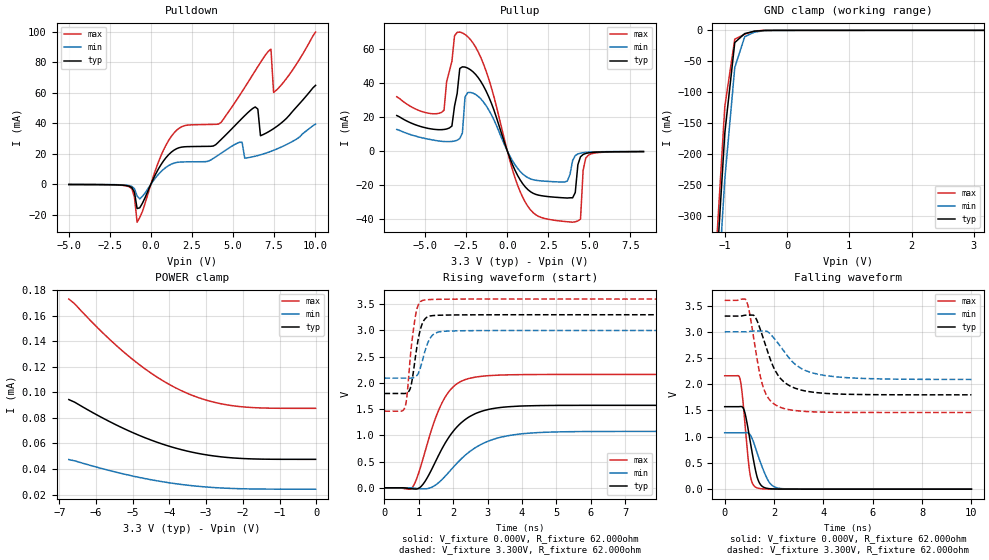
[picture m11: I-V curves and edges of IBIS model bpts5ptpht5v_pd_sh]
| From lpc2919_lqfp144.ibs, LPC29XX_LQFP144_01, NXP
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| |   Rev 0.20 IBIS Model Design Automation Generation   |
| |   N O N - S I L I C O N   C O R R E L A T E D   |
| |   This IBIS [Model] is pre-Beta tactical support   |
| |  Note: this IBIS [Model] contains clamp curves generated   |
| |   through simulation which should not be relied upon   |
| Pccmos14 hliolib_nlm 4.0.1
|   0.18 um 3.3V pad library
|   six level metal
|   dual oxide
|   single threshold voltage
|   nominal line mixed supply
|   parasitic extracted netlists
| Process block c14
| bpts5ptpht5v
|   Bidirectional Pad 3v3
|   3state Output
|   Plain Input
|   1ns Slew Rate control
|   CMOS
|   Programmable between
|   - (p1=0, p2=1) plain input
|   - (p1=0, p2=0) with Pull Up
|   - (p1=1, p2=1) with Pull Down
|   - (p1=1, p2=0) with Repeater
|   Characterized at Core 1.8V and I/O 3.3V
| Pull Down Mode (p1=1, p2=1)
[Model]   bpts5ptpht5v_pd_sh | of bpts5ptpht5v
Model_type   I/O
Polarity   Non-Inverting
Enable   Active-Low
|  Reciever Thresholds
Vinl   = 0.99V
Vinh   = 2.31V
| AC Test Load Conditions
Vref   = 0
Cref   = 1.2e-11
Rref   = 1000000000
Vmeas   = 1.65
| [Process Range]   typical   min   max
| C_comp edge width   400.000ps   400.000ps   400.000ps
| C_comp Tstrobe   40.000fs   40.000fs   40.000fs
C_comp   2.521pF   2.386pF   2.657pF
[Temperature Range]   25   125   -40
[Voltage Range]   3.30V   3.00V   3.60V
[GND Clamp Reference]   0.00V   0.00V   0.00V
[Pulldown Reference]   0.00V   0.00V   0.00V
[POWER Clamp Reference]   3.30V   3.00V   3.60V
[Pullup Reference]   3.30V   3.00V   3.60V
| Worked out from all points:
|   slope of the pulldown table from 0 to 0.495 V, typ, clamps not added: 46.5 ohm
|   slope of the pullup table from 0 to 0.495 V, typ, clamps not added: 41.9 ohm
|   GND clamp passes 1 mA (typ) near -0.48 V on its own axis
|   rising waveform, V_fixture 0.000V, R_fixture 62.000ohm: 20-80 % time 921ps typ, 1.16ns min, 700ps max; typ from 0 V to 1.57 V
|   falling waveform, V_fixture 0.000V, R_fixture 62.000ohm: 20-80 % time 364ps typ, 508ps min, 256ps max; typ from 1.57 V to 0 V
|   rising waveform, V_fixture 3.300V, R_fixture 62.000ohm: 20-80 % time 223ps typ, 262ps min, 202ps max; typ from 1.8 V to 3.3 V
|   falling waveform, V_fixture 3.300V, R_fixture 62.000ohm: 20-80 % time 809ps typ, 1.12ns min, 527ps max; typ from 3.3 V to 1.8 V
[GND Clamp]
| ref voltage   0.00V   0.00V   0.00V
|   Voltage   I(typ)   I(min)   I(max)
-5V       -7.933A    -7.953A    -7.929A
-1.16V    -429.6mA   -501mA     -389.4mA
-1V       -166mA     -240.8mA   -123.1mA
-840mV    -19.71mA   -60.08mA   -14.11mA
-680mV    -5.172mA   -10.16mA   -6.119mA
-520mV    -1.294mA   -2.638mA   -834.5uA
-200mV    -15.34uA   -18.05uA   -23.66uA
3.16V     47.55uA    24.23uA    87.44uA
[Power Clamp]   | Vtable = Vcc - Vpad
| ref voltage   3.30V   3.00V   3.60V
|   Voltage   I(typ)   I(min)   I(max)
-6.74V    94.28uA    47.4uA     172.9uA
-6.58V    92.21uA    46.36uA    169.1uA
-6.1V     84.26uA    42.38uA    154.6uA
-5.62V    76.9uA     38.71uA    141.1uA
-4.98V    68.19uA    34.37uA    125.2uA
-4.5V     62.6uA     31.59uA    114.9uA
-4.18V    59.37uA    29.99uA    109uA
-3.54V    54.16uA    27.42uA    99.49uA
-2.9V     50.63uA    25.7uA     93.05uA
-2.26V    48.64uA    24.74uA    89.4uA
-1.46V    47.7uA     24.3uA     87.7uA
-20mV     47.55uA    24.23uA    87.44uA
[Pulldown]
| ref voltage   0.00V   0.00V   0.00V
|   Voltage   I(typ)   I(min)   I(max)
-5V       -187.5uA   -145.7uA   -211.8uA
-1.32V    -1.32mA    -939.4uA   -1.723mA
-1V       -5.322mA   -2.96mA    -8.616mA
-840mV    -15.95mA   -7.733mA   -24.9mA
1.4V      22.26mA    13.79mA    33.48mA
4.28V     29.29mA    20.29mA    40.56mA
5.56V     43.21mA    27.48mA    60.71mA
6.36V     50.65mA    18.36mA    74.35mA
6.68V     31.77mA    19.27mA    79.79mA
7.32V     35.33mA    21.55mA    88.5mA
7.48V     36.43mA    22.22mA    60.17mA
10.04V    64.8mA     39.39mA    99.71mA
[Pullup]   | Vtable = Vcc - Vpad
| ref voltage   3.30V   3.00V   3.60V
|   Voltage   I(typ)   I(min)   I(max)
-6.74V    20.77mA    12.63mA    31.77mA
-3.86V    12.61mA    5.565mA    23.86mA
-3.22V    26.24mA    5.844mA    67.45mA
-2.74V    49.27mA    10.56mA    69.13mA
-2.58V    49.14mA    31.6mA     68.22mA
780mV     -16.88mA   -11.92mA   -23.75mA
2.38V     -26.56mA   -17.72mA   -39.7mA
3.98V     -27.38mA   -5.509mA   -41.66mA
4.46V     -3.36mA    -1.235mA   -39.9mA
4.62V     -2.02mA    -961.4uA   -11.27mA
4.94V     -1.105mA   -662.3uA   -2.417mA
8.3V      -310.5uA   -276uA     -365.2uA
[Ramp]
R_load   = 62.000ohm
|   dV/dt(typ)   dV/dt(min)   dV/dt(max)
dV/dt_r   722.040mV/915.000ps   485.123mV/1.125ns   1.049V/765.000ps
dV/dt_f   679.651mV/810.000ps   405.014mV/1.100ns   1.042V/590.000ps
[Rising Waveform]  | cubic spline decimation from 2001 points
V_fixture   = 0.000V
R_fixture   = 62.000ohm
|   Time   V(typ)   V(min)   V(max)
0s        2.032nV    363.7nV    1.043nV
820ps     -20.77mV   -5.722mV   13.87mV
1.15ns    91.74mV    -19.9mV    616.1mV
1.45ns    450.3mV    36.17mV    1.263V
1.655ns   719.3mV    144.1mV    1.591V
2.01ns    1.084V     396.8mV    1.93V
2.38ns    1.315V     636.8mV    2.069V
3.12ns    1.506V     913mV      2.141V
4.09ns    1.561V     1.035V     2.158V
10ns      1.572V     1.075V     2.161V
[Falling Waveform]  | cubic spline decimation from 2001 points
V_fixture   = 0.000V
R_fixture   = 62.000ohm
|   Time   V(typ)   V(min)   V(max)
0s        1.572V     1.075V     2.161V
620ps     1.574V     1.075V     2.104V
795ps     1.495V     1.076V     1.391V
1.015ns   961.7mV    1.047V     321.8mV
1.115ns   689.4mV    961.8mV    122.8mV
1.29ns    274.3mV    727.3mV    29.15mV
1.47ns    76.73mV    483.5mV    9.363mV
1.755ns   12.7mV     169.2mV    2.954mV
2.185ns   2.64mV     19.15mV    1.23mV
10ns      415.3nV    6.218uV    21.21nV
[Rising Waveform]  | cubic spline decimation from 2001 points
V_fixture   = 3.300V
V_fixture_min = 3.000V
V_fixture_max = 3.600V
R_fixture   = 62.000ohm
|   Time   V(typ)   V(min)   V(max)
0s        1.798V     2.091V     1.461V
600ps     1.798V     2.091V     1.543V
650ps     1.807V     2.091V     1.721V
755ps     1.901V     2.091V     2.508V
890ps     2.437V     2.112V     3.224V
980ps     2.822V     2.175V     3.479V
1.1ns     3.127V     2.412V     3.569V
1.34ns    3.277V     2.862V     3.589V
1.67ns    3.291V     2.98V      3.594V
10ns      3.299V     2.999V     3.598V
[Falling Waveform]  | cubic spline decimation from 2001 points
V_fixture   = 3.300V
V_fixture_min = 3.000V
V_fixture_max = 3.600V
R_fixture   = 62.000ohm
|   Time   V(typ)   V(min)   V(max)
0s        3.299V     2.999V     3.598V
880ps     3.317V     3V         3.587V
1.005ns   3.318V     3.006V     3.367V
1.19ns    3.307V     3.014V     2.837V
1.54ns    2.909V     3.013V     1.975V
1.815ns   2.52V      2.974V     1.706V
2.155ns   2.175V     2.785V     1.58V
2.87ns    1.921V     2.374V     1.498V
3.81ns    1.836V     2.188V     1.47V
10ns      1.798V     2.091V     1.461V
